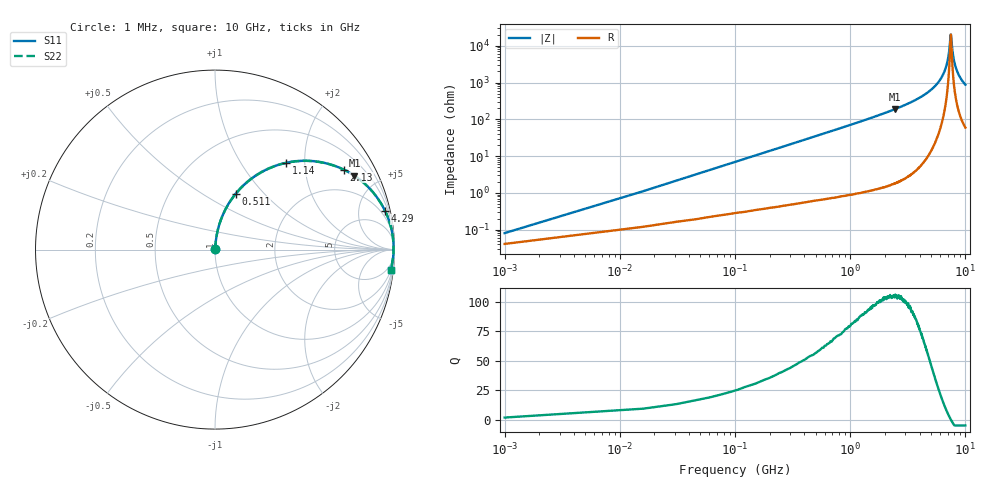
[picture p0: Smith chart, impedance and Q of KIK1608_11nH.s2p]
!version-2
!date-01.2022
!Series
# MHz S RI R 50
!Freq ReS11 ImS11 ReS21 ImS21 ReS12 ImS12 ReS22 ImS22
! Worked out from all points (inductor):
!   668 points, 1 MHz to 10 GHz, reference 50 ohm
!   read as one part in series: L = 11 nH near 46 MHz
!   highest Q = 105 at 2.43 GHz (marker M1), where L = 12.3 nH
!   self-resonance near 7.47 GHz
!   S11 on the Smith chart (normalised r, x): 1 MHz: 1.00, +0.00; 511 MHz: 1.01, +0.71; 1.14 GHz: 1.02, +1.61; 2.13 GHz: 1.03, +3.21; 4.29 GHz: 1.13, +8.85; 10 GHz: 2, -17
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1  0.000416 0.000691  0.9996 -0.000691  0.9996 -0.000691  0.000416 0.000691
61  0.00397 0.0419  0.996 -0.0419  0.996 -0.0419  0.00397 0.0419
121  0.00993 0.0826  0.9901 -0.0826  0.9901 -0.0826  0.00993 0.0826
271  0.038 0.1796  0.962 -0.1796  0.962 -0.1796  0.038 0.1796
511  0.1161 0.3117  0.8839 -0.3117  0.8839 -0.3117  0.1161 0.3117
1140  0.3959 0.4832  0.6041 -0.4832  0.6041 -0.4832  0.3959 0.4832
1670  0.5939 0.486  0.4061 -0.486  0.4061 -0.486  0.5939 0.486
2130  0.718 0.4452  0.282 -0.4452  0.282 -0.4452  0.718 0.4452
2430  0.7771 0.4114  0.2229 -0.4114  0.2229 -0.4114  0.7771 0.4114
3350  0.8907 0.3068  0.1093 -0.3068  0.1093 -0.3068  0.8907 0.3068
4290  0.9486 0.2137  0.0514 -0.2137  0.0514 -0.2137  0.9486 0.2137
5010  0.9722 0.154  0.0278 -0.154  0.0278 -0.154  0.9722 0.154
5990  0.9888 0.0853  0.0112 -0.0853  0.0112 -0.0853  0.9888 0.0853
6680  0.9939 0.0433  0.00613 -0.0433  0.00613 -0.0433  0.9939 0.0433
7130  0.9951 0.0183  0.00493 -0.0183  0.00493 -0.0183  0.9951 0.0183
7470  0.9951 0.000141  0.00489 -0.000141  0.00489 -0.000141  0.9951 0.000141
7520  0.9951 -0.00216  0.00494 0.00216  0.00494 0.00216  0.9951 -0.00216
7680  0.9948 -0.0105  0.0052 0.0105  0.0052 0.0105  0.9948 -0.0105
7860  0.9944 -0.0193  0.00564 0.0193  0.00564 0.0193  0.9944 -0.0193
8340  0.9925 -0.042  0.00753 0.042  0.00753 0.042  0.9925 -0.042
9030  0.9882 -0.0723  0.0118 0.0723  0.0118 0.0723  0.9882 -0.0723
10000  0.9796 -0.1111  0.0204 0.1111  0.0204 0.1111  0.9796 -0.1111
